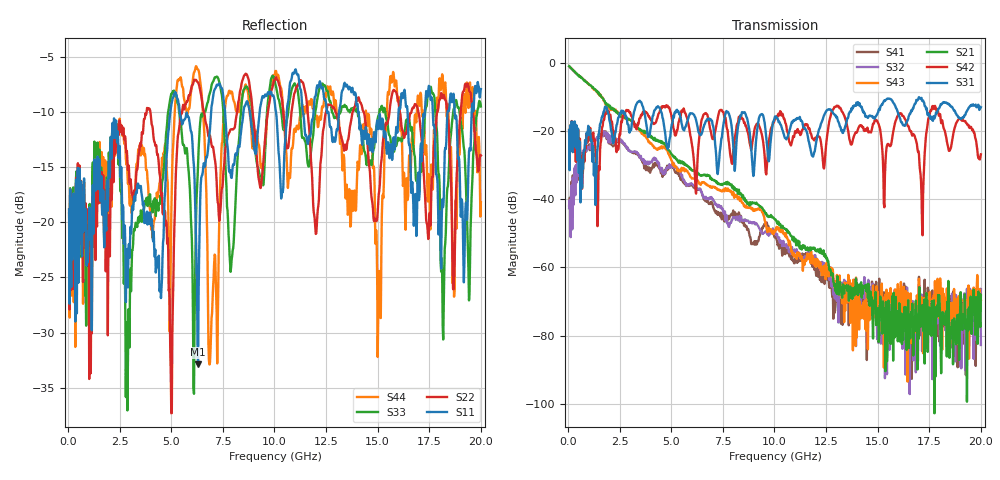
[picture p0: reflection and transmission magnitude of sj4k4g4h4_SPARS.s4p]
! FILE: E:\users\goganessyan\GBX_Backplane\FR408_backplane\1m_INBOUND_TRU\sj4k4g4h4_SPARS.s4p
# MHZ S RI R 50.00
! FREQ  S11  S12  S13  S14
!  S21  S22  S23  S24
!  S31  S32  S33  S34
!  S41  S42  S43  S44
!  REAL  IMAG  REAL  IMAG  REAL  IMAG  REAL  IMAG
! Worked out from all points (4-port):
!   799 points, 50 MHz to 20 GHz, reference 50 ohm
!   strongest paths, dB at 50 MHz, 5.025 GHz, 10.03 GHz, 15.03 GHz, 20 GHz:
!     S31: -19.8, -18.1, -15.8, -14.5, -13.1
!     S42: -19.7, -16.4, -16.7, -17.8, -26.9
!     S21: -1.0, -26.9, -46.0, -71.9, -68.1
!     S43: -1.1, -28.8, -49.6, -72.0, -69.5
!     S32: -42.7, -29.8, -49.5, -82.1, -82.7
!     S41: -41.8, -30.1, -51.3, -66.4, -66.4
!   lowest |S11| = -32.9 dB at 6.3 GHz (marker M1), VSWR 1.05, Z = 48.5 - j1.62 ohm
!   |S11| at or under -10 dB: start of sweep to 4.96 GHz; 5.41 GHz to 6.93 GHz (1.521 GHz wide, 24.6 % of centre); 14.08 GHz to 16.01 GHz (1.938 GHz wide, 12.9 % of centre)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
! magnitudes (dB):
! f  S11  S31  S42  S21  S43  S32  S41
! 50 MHz  -18.9  -19.8  -19.7  -1.0  -1.1  -42.7  -41.8
! 3.9 GHz  -19.1  -21.5  -15.7  -21.0  -23.3  -29.5  -31.8
! 5 GHz  -9.4  -19.0  -15.3  -26.7  -28.5  -30.3  -30.1
! 6.3 GHz  -32.9  -19.8  -25.6  -32.4  -34.7  -37.0  -37.2
! 6.875 GHz  -11.6  -16.9  -19.2  -33.5  -36.1  -39.8  -41.0
! 7.85 GHz  -15.3  -16.1  -26.6  -35.7  -37.8  -46.8  -44.9
! 20 GHz  -7.9  -13.1  -26.9  -68.1  -69.5  -82.7  -66.4
